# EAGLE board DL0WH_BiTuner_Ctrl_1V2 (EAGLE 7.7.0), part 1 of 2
DL0WH Antenna BiTuner
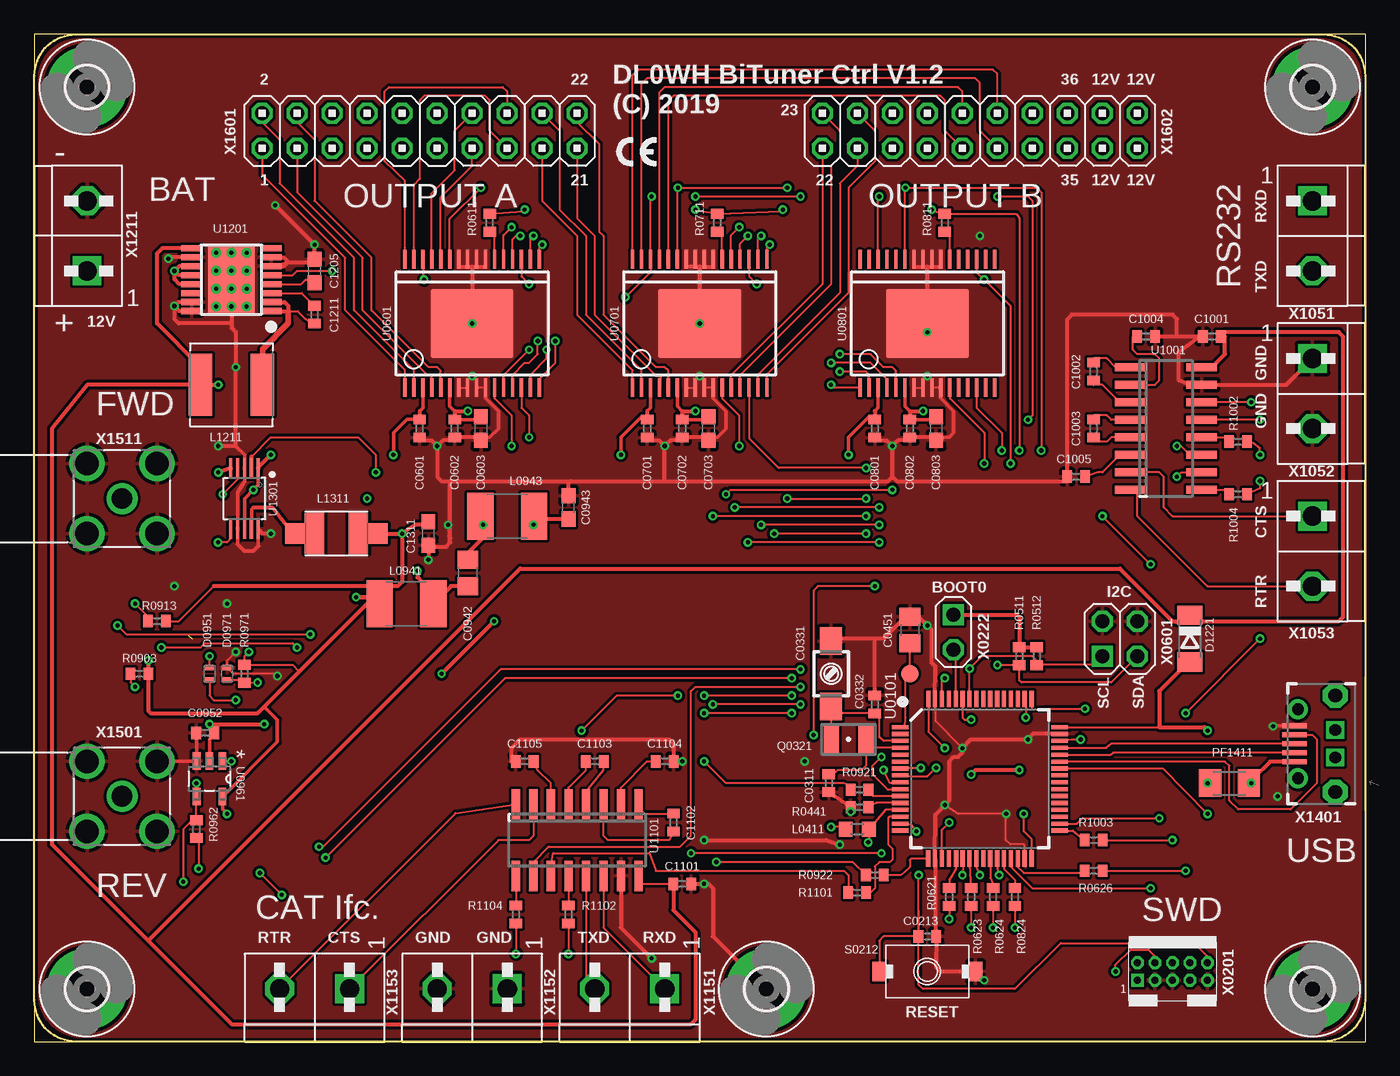
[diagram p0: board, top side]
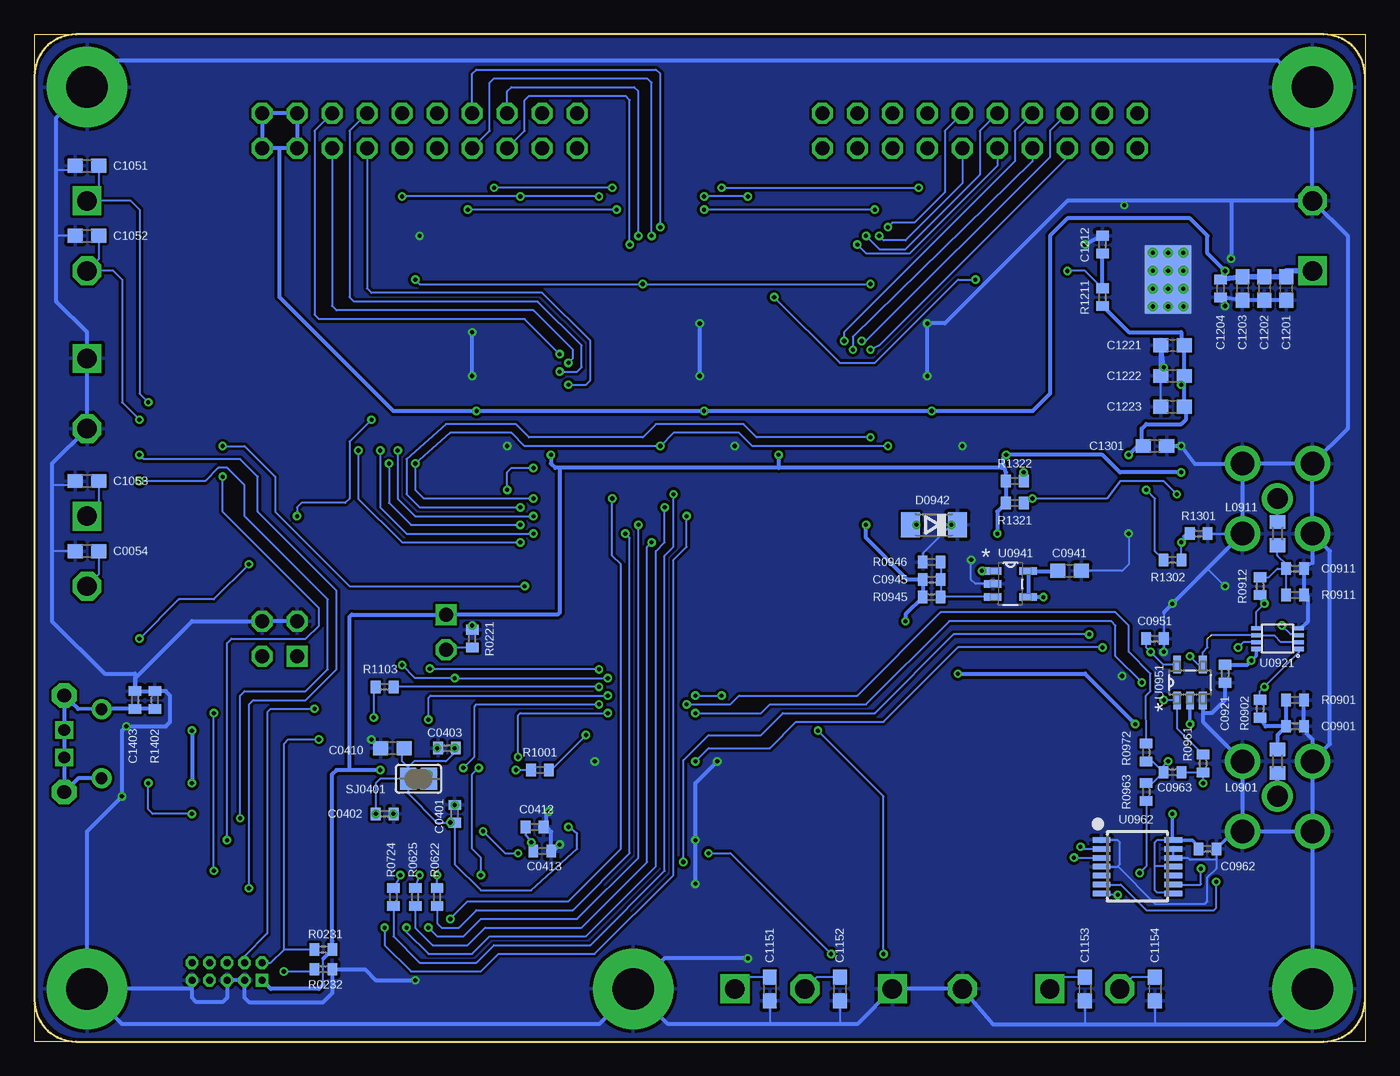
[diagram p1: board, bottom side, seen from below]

Size 96.52 x 73.03 mm. Coordinates in mm from the lower left corner, seen from the top.
Outline: 0,0 96.52,0 96.52,73.03 0,73.03 0,0
Copper layers (1*16): Top 0.035mm / dielectric 1.5mm / Bottom 0.035mm
Design rules "DL0WH_BiTuner_MCU_1V2": minimum track width 6mil, minimum drill 0.3mm, track to track 8mil, track to pad 8mil, pad to pad 6mil, via to via 8mil, smd to smd 0mil, copper to edge 10mil, drill to drill 10mil, minimum pad ring 8mil, minimum via ring 6mil, stop-mask expansion 2mil, vias tented up to drill 25mil, thermal gap 10mil
Net classes: 1 pwr_relay: width 1.5 mm, clearance 0.5 mm; 2 pwr_ttl: width 0.75 mm, clearance 0.5 mm; 3 usb_pair: width 0.254 mm, clearance 0.152 mm; 4 pwrA5: width 0.4 mm; 5 single50R: width 0.838 mm, clearance 0.152 mm; 6 mil6_nofill: width 0.152 mm, clearance 0.254 mm
Milling: 8 lines

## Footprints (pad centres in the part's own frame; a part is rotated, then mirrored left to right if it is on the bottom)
C0603 = smd 1.1 x 1: 1 -0.85,0; 2 0.85,0
C0402 = smd 0.7 x 0.9: 1 -0.65,0; 2 0.65,0
3MM2_X_2MM5 = smd 2 x 1.6: + -2.365,0; - 2.365,0
C0805 = smd 1.3 x 1.5: 1 -0.95,0; 2 0.95,0
SOD80C = smd 1.4 x 1.8: A 1.7,0; C -1.7,0
SOD923 = smd 0.4 x 0.6: A 0.45,0; C -0.45,0
3,0-PAD = drill 3 pad 5.842: B3,0 0,0
L0603 = smd 1 x 1.1: 1 -0.85,0; 2 0.85,0
L1812 = smd 1.9 x 3.4: 1 -1.95,0; 2 1.95,0
L_6.00MM_X_6.00MM = smd 1.7 x 4.5: 1 -2.25,0; 2 2.25,0
L_4.50MM_X_3.20MM = smd 1.5 x 3: 1 -1.6,0; 2 1.6,0 | smd 2 x 1.5: 3 -2.75,0; 4 2.75,0
M1206 = smd 1.6 x 2: 1 -1.4,0; 2 1.4,0
ABS07 = smd 1.1 x 1.9: 1 -1.25,0; 2 1.25,0
R0402 = smd 0.7 x 0.9: 1 -0.65,0; 2 0.65,0
KSR223G_SMD_1POL = smd 1 x 1.4: 1 -3.5,0; 2 3.5,0
SJ = smd 1.168 x 1.6: 1 -0.762,0; 2 0.762,0
B1,27 = smd 1.27 x 1.27: TP 0,0
LQFP64 = smd 1.2 x 0.3: 1 -5.775,3.75; 2 -5.775,3.25; 3 -5.775,2.75; 4 -5.775,2.25; 5 -5.775,1.75; 6 -5.775,1.25; 7 -5.775,0.75; 8 -5.775,0.25; 9 -5.775,-0.25; 10 -5.775,-0.75; 11 -5.775,-1.25; 12 -5.775,-1.75; 13 -5.775,-2.25; 14 -5.775,-2.75; 15 -5.775,-3.25; 16 -5.775,-3.75; 33 5.775,-3.75; 34 5.775,-3.25; 35 5.775,-2.75; 36 5.775,-2.25; 37 5.775,-1.75; 38 5.775,-1.25; 39 5.775,-0.75; 40 5.775,-0.25; 41 5.775,0.25; 42 5.775,0.75; 43 5.775,1.25; 44 5.775,1.75; 45 5.775,2.25; 46 5.775,2.75; 47 5.775,3.25; 48 5.775,3.75 | smd 0.3 x 1.2: 17 -3.75,-5.775; 18 -3.25,-5.775; 19 -2.75,-5.775; 20 -2.25,-5.775; 21 -1.725,-5.775; 22 -1.25,-5.775; 23 -0.75,-5.775; 24 -0.25,-5.775; 25 0.25,-5.775; 26 0.75,-5.775; 27 1.25,-5.775; 28 1.75,-5.775; 29 2.25,-5.775; 30 2.75,-5.775; 31 3.25,-5.775; 32 3.75,-5.775; 49 3.75,5.775; 50 3.25,5.775; 51 2.75,5.775; 52 2.25,5.775; 53 1.75,5.775; 54 1.25,5.775; 55 0.75,5.775; 56 0.25,5.775; 57 -0.25,5.775; 58 -0.75,5.775; 59 -1.25,5.775; 60 -1.75,5.775; 61 -2.25,5.775; 62 -2.75,5.775; 63 -3.25,5.775; 64 -3.725,5.775
SOICW32 = smd 0.25 x 1.3: 1 -4.875,-4.65; 2 -4.225,-4.65; 3 -3.575,-4.65; 4 -2.925,-4.65; 5 -2.275,-4.65; 6 -1.625,-4.65; 7 -0.975,-4.65; 8 -0.325,-4.65; 9 0.325,-4.65; 10 0.975,-4.65; 11 1.625,-4.65; 12 2.275,-4.65; 13 2.925,-4.65; 14 3.575,-4.65; 15 4.225,-4.65; 16 4.875,-4.65; 17 4.875,4.65; 18 4.225,4.65; 19 3.575,4.65; 20 2.925,4.65; 21 2.275,4.65; 22 1.625,4.65; 23 0.975,4.65; 24 0.325,4.65; 25 -0.325,4.65; 26 -0.975,4.65; 27 -1.625,4.65; 28 -2.275,4.65; 29 -2.925,4.65; 30 -3.575,4.65; 31 -4.225,4.65; 32 -4.875,4.65 | smd 6 x 5: 33 0,0
R-PDSO-G8 = smd 0.25 x 0.75: 1 -0.75,-1.55; 2 -0.25,-1.55; 3 0.25,-1.55; 4 0.75,-1.55; 5 0.75,1.55; 6 0.25,1.55; 7 -0.25,1.55; 8 -0.75,1.55
SOT95P280X145-5N = smd 1.27 x 0.559: 1 -1.295,0.94; 2 -1.295,0; 3 -1.295,-0.94; 4 1.295,-0.94; 5 1.295,0.94
SOT-23-5 = smd 1.27 x 0.559: 1 -1.295,0.94; 2 -1.295,0; 3 -1.295,-0.94; 4 1.295,-0.94; 5 1.295,0.94
TSSOP14 = smd 0.4 x 1.3: 1 -1.925,-2.6; 2 -1.275,-2.6; 3 -0.625,-2.6; 4 0.025,-2.6; 5 0.675,-2.6; 6 1.325,-2.6; 7 1.975,-2.6; 8 1.975,2.6; 9 1.325,2.6; 10 0.675,2.6; 11 0.025,2.6; 12 -0.625,2.6; 13 -1.275,2.6; 14 -1.925,2.6
SOIC16N = smd 0.6 x 2.2: 1 -4.445,-2.6; 2 -3.175,-2.6; 3 -1.905,-2.6; 4 -0.635,-2.6; 5 0.635,-2.6; 6 1.905,-2.6; 7 3.175,-2.6; 8 4.445,-2.6; 9 4.445,2.6; 10 3.175,2.6; 11 1.905,2.6; 12 0.635,2.6; 13 -0.635,2.6; 14 -1.905,2.6; 15 -3.175,2.6; 16 -4.445,2.6
HTSSOP16 = smd 0.45 x 1.5: 1 -2.275,-2.9; 2 -1.625,-2.9; 3 -0.975,-2.9; 4 -0.325,-2.9; 5 0.325,-2.9; 6 0.975,-2.9; 7 1.625,-2.9; 8 2.275,-2.9; 9 2.275,2.9; 10 1.625,2.9; 11 0.975,2.9; 12 0.325,2.9; 13 -0.325,2.9; 14 -0.975,2.9; 15 -1.625,2.9; 16 -2.275,2.9 | drill 0.305 pad 0.61: PAD 0.65,0; PAD3 -0.65,0; PAD4 -1.95,0; PAD5 1.95,0; PAD6 1.95,1.1; PAD7 1.95,-1.1; PAD8 0.65,1.1; PAD9 0.65,-1.1; PAD10 -0.65,1.1; PAD11 -0.65,-1.1; PAD12 -1.95,1.1; PAD13 -1.95,-1.1 | smd 5 x 3.4: PAD1 0,0 | smd 5 x 3.4 bottom: PAD2 0,0
S-PDSO-G10 = smd 0.3 x 1.45: 1 -1,-2.2; 2 -0.5,-2.2; 3 0,-2.2; 4 0.5,-2.2; 5 1,-2.2; 6 1,2.2; 7 0.5,2.2; 8 0,2.2; 9 -0.5,2.2; 10 -1,2.2
2X05_1MM27_SHROUDED_CORTEX_JTAG_SWD = drill 0.5 pad 0.914 square: 1 -2.54,-0.635 | drill 0.5 pad 0.914 octagon: 2 -2.54,0.635; 3 -1.27,-0.635; 4 -1.27,0.635; 5 0,-0.635; 6 0,0.635; 7 1.27,-0.635; 8 1.27,0.635; 9 2.54,-0.635; 10 2.54,0.635
1X02 = drill 1.016 square: 1 0,0 | drill 1.016 octagon: 2 0,2.54
2X02 = drill 1.016 square: 1 -1.27,-1.27 | drill 1.016 octagon: 2 -1.27,1.27; 3 1.27,-1.27; 4 1.27,1.27
WIRE-TO-BOARD_5MM08_1X02 = drill 1.4 square: 1 0,2.54 | drill 1.4 octagon: 2 0,-2.54
USB-B-MICRO-SMD_MOLEX-105017-0001 = smd 0.35 x 1.8: D+ 0,4.4; D- -0.65,4.4; GND 1.3,4.4; ID 0.65,4.4; VBUS -1.3,4.4 | drill 0.85 pad 1.45: JSHIELD -2.5,4.15; JSHIELD@2 2.5,4.15 | drill 1 pad 1.8 octagon: JSHIELD@3 -3.5,1.45; JSHIELD@6 3.5,1.45 | drill 0.85 square: JSHIELD@4 -1,1.45; JSHIELD@5 1,1.45
SMA_SMT_AMPHENOL_901-143 = drill 1.499: 1 0,0 | drill 1.702: 2 -2.54,2.54; 3 -2.54,-2.54; 4 2.54,-2.54; 5 2.54,2.54
2X10 = drill 1.016 octagon: 1 -11.43,-1.27; 2 -11.43,1.27; 3 -8.89,-1.27; 4 -8.89,1.27; 5 -6.35,-1.27; 6 -6.35,1.27; 7 -3.81,-1.27; 8 -3.81,1.27; 9 -1.27,-1.27; 10 -1.27,1.27; 11 1.27,-1.27; 12 1.27,1.27; 13 3.81,-1.27; 14 3.81,1.27; 15 6.35,-1.27; 16 6.35,1.27; 17 8.89,-1.27; 18 8.89,1.27; 19 11.43,-1.27; 20 11.43,1.27

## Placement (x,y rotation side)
C0054  10nF  [C0603]  92.71,35.56 180 bottom
C0213  100nF  [C0402]  64.77,7.62 0 top
C0311  22pF  [C0402]  57.63,18.73 270 top
C0331  JR200  [3MM2_X_2MM5]  57.78,26.67 270 top
C0332  18pF  [C0402]  60.96,24.45 90 top
C0401  100nF  [C0402]  66.04,16.51 90 bottom
C0402  100nF  [C0402]  71.12,16.51 0 bottom
C0403  100nF  [C0402]  66.6,21.27 180 bottom
C0410  4.7uF  [C0603]  70.56,21.27 180 bottom
C0412  10nF  [C0402]  60.25,15.56 0 bottom
C0413  1uF  [C0402]  59.69,13.81 0 bottom
C0451  47uF  [C0805]  63.5,29.84 90 top
C0601  100nF  [C0402]  27.94,44.45 90 top
C0602  100nF  [C0402]  30.48,44.45 270 top
C0603  22uF  [C0603]  32.38,44.45 270 top
C0701  100nF  [C0402]  44.45,44.45 90 top
C0702  100nF  [C0402]  46.99,44.45 270 top
C0703  22uF  [C0603]  48.9,44.45 270 top
C0801  100nF  [C0402]  60.96,44.45 90 top
C0802  100nF  [C0402]  63.5,44.45 270 top
C0803  22uF  [C0603]  65.41,44.45 270 top
C0901  1nF  [C0402]  5.08,22.86 0 bottom
C0911  1nF  [C0402]  5.08,34.29 0 bottom
C0921  100nF  [C0402]  10.16,26.67 270 bottom
C0941  22uF  [C0603]  21.43,34.13 0 bottom
C0942  2.2uF  [C0805]  31.43,33.97 90 top
C0943  22uF  [C0603]  38.73,38.73 90 top
C0945  1nF  [C0402]  31.43,33.5 180 bottom
C0951  100nF  [C0402]  15.24,29.21 0 bottom
C0952  100nF  [C0402]  12.38,22.38 180 top
C0962  100nF  [C0402]  11.43,13.97 0 bottom
C0963  100pF  [C0402]  13.97,19.53 180 bottom
C1001  1uF  [C0402]  85.41,51.12 180 top
C1002  1uF  [C0402]  76.83,48.58 270 top
C1003  1uF  [C0402]  76.83,44.45 270 top
C1004  1uF  [C0402]  80.64,51.12 0 top
C1005  1uF  [C0402]  75.56,40.96 180 top
C1051  10nF  [C0603]  92.71,63.5 180 bottom
C1052  10nF  [C0603]  92.71,58.42 180 bottom
C1053  10nF  [C0603]  92.71,40.64 180 bottom
C1101  1uF  [C0402]  46.99,11.43 0 top
C1102  1uF  [C0402]  46.35,15.88 270 top
C1103  1uF  [C0402]  40.64,20.32 180 top
C1104  1uF  [C0402]  45.72,20.32 0 top
C1105  1uF  [C0402]  35.56,20.32 180 top
C1151  10nF  [C0603]  43.18,3.81 270 bottom
C1152  10nF  [C0603]  38.1,3.81 270 bottom
C1153  10nF  [C0603]  20.32,3.81 270 bottom
C1154  10nF  [C0603]  15.24,3.81 270 bottom
C1201  10uF  [C0603]  5.71,54.61 270 bottom
C1202  10uF  [C0603]  7.3,54.61 270 bottom
C1203  10uF  [C0603]  8.89,54.61 270 bottom
C1204  10nF  [C0402]  10.48,54.61 270 bottom
C1205  3.3uF  [C0603]  20.32,55.88 270 top
C1211  0.47uF  [C0402]  20.32,52.7 90 top
C1212  100nF  [C0402]  19.05,57.78 90 bottom
C1221  22uF  [C0603]  13.97,50.48 180 bottom
C1222  22uF  [C0603]  13.97,48.26 180 bottom
C1223  22uF  [C0603]  13.97,46.04 180 bottom
C1301  22uF  [C0603]  15.24,43.18 0 bottom
C1311  22uF  [C0603]  28.57,36.83 270 top
C1403  1nF  [C0402]  89.22,24.77 270 bottom
D0942  CRS08  [SOD80C]  31.27,37.47 180 bottom
D0951  CMAD6001  [SOD923]  12.7,26.67 90 top
D0971  CMAD6001  [SOD923]  13.97,26.67 270 top
D1221  CRS08  [SOD80C]  83.82,29.21 270 top
H1711  MOUNT-PAD-ROUND3.0  [3,0-PAD]  3.81,3.81 0 top
H1721  MOUNT-PAD-ROUND3.0  [3,0-PAD]  53.09,3.81 0 top
H1731  MOUNT-PAD-ROUND3.0  [3,0-PAD]  92.71,3.81 0 top
H1751  MOUNT-PAD-ROUND3.0  [3,0-PAD]  3.81,69.22 0 top
H1761  MOUNT-PAD-ROUND3.0  [3,0-PAD]  92.71,69.22 0 top
L0411  10uH  [L0603]  59.69,15.4 0 top
L0901  10uH  [L0603]  6.35,20.32 270 bottom
L0911  10uH  [L0603]  6.35,36.83 90 bottom
L0941  20uH  [L1812]  26.99,31.75 180 top
L0943  20uH  [L1812]  34.29,38.1 180 top
L1211  2.2uH  [L_6.00MM_X_6.00MM]  14.29,47.62 0 top
L1311  10uH  [L_4.50MM_X_3.20MM]  21.91,36.83 180 top
PF1411  1.1A/2.2A  [M1206]  86.68,18.73 180 top
Q0321  ABS07-32.768KHZ  [ABS07]  59.05,21.91 180 top
R0221  33kR  [R0402]  64.77,29.21 270 bottom
R0231  220kR  [R0402]  75.56,6.67 0 bottom
R0232  220kR  [R0402]  75.56,5.24 180 bottom
R0441  0R  [R0402]  59.85,16.99 0 top
R0511  1kR  [R0402]  71.44,27.94 90 top
R0512  1kR  [R0402]  72.71,27.94 90 top
R0611  47R  [R0402]  33.02,59.37 270 top
R0621  47R  [R0402]  66.36,10.48 270 top
R0622  0R  [R0402]  67.31,10.48 270 bottom
R0623  47R  [R0402]  67.94,10.48 270 top
R0624  47R  [R0402]  69.53,10.48 270 top
R0625  47R  [R0402]  68.9,10.48 270 bottom
R0626  47R  [R0402]  76.83,12.38 0 top
R0711  47R  [R0402]  49.53,59.37 270 top
R0724  47R  [R0402]  70.48,10.48 270 bottom
R0811  47R  [R0402]  66.04,59.37 270 top
R0824  47R  [R0402]  71.12,10.48 270 top
R0901  1kR  [R0402]  5.08,24.77 180 bottom
R0902  15kR  [R0402]  7.62,24.13 90 bottom
R0903  150kR  [R0402]  7.62,26.67 0 top
R0911  1kR  [R0402]  5.08,32.38 180 bottom
R0912  15kR  [R0402]  7.62,33.02 270 bottom
R0913  150kR  [R0402]  8.89,30.48 0 top
R0921  47R  [R0402]  59.85,18.26 180 top
R0922  47R  [R0402]  60.96,12.06 180 top
R0945  8.2kR  [R0402]  31.43,32.23 180 bottom
R0946  33kR  [R0402]  31.43,34.77 0 bottom
R0961  1kR  [R0402]  11.75,20.16 270 bottom
R0962  1.0kR  [R0402]  11.75,15.4 270 top
R0963  10kR  [R0402]  15.88,18.1 90 bottom
R0971  10kR  [R0402]  15.24,26.67 270 top
R0972  47R  [R0402]  15.88,20.95 90 bottom
R1001  47R  [R0402]  59.85,19.68 0 bottom
R1002  47R  [R0402]  87.31,43.5 180 top
R1003  47R  [R0402]  76.83,14.61 0 top
R1004  47R  [R0402]  87.31,39.69 180 top
R1101  47R  [R0402]  59.69,10.79 180 top
R1102  47R  [R0402]  38.73,9.21 90 top
R1103  47R  [R0402]  71.12,25.72 0 bottom
R1104  47R  [R0402]  34.92,9.21 90 top
R1211  3R  [R0402]  19.05,53.98 270 bottom
R1301  100kR  [R0402]  12.06,36.83 180 bottom
R1302  220kR  [R0402]  13.97,34.92 180 bottom
R1321  1MR  [R0402]  25.4,39.05 180 bottom
R1322  1MR  [R0402]  25.4,40.64 180 bottom
R1402  330kR  [R0402]  87.79,24.77 270 bottom
S0212  KSR223GLFG  [KSR223G_SMD_1POL]  64.77,5.08 180 top
SJ0401  [SJ]  68.66,19.05 180 bottom
TP_VBAT  PTR1B1,27  [B1,27]  63.5,26.67 0 top
U0101  STM32L476RXT_64PIN_LDO  [LQFP64]  68.58,19.05 0 top
U0601  MC33996  [SOICW32]  31.75,52.07 0 top
U0701  MC33996  [SOICW32]  48.26,52.07 0 top
U0801  MC33996  [SOICW32]  64.77,52.07 0 top
U0921  TS5A23166  [R-PDSO-G8]  6.35,29.21 90 bottom
U0941  LM2611  [SOT95P280X145-5N]  25.72,33.18 0 bottom
U0951  OPA354  [SOT-23-5]  12.7,26.04 90 bottom
U0961  OPA354  [SOT-23-5]  12.7,19.05 270 top
U0962  MCP4661-103E-MS  [TSSOP14]  16.51,12.7 270 bottom
U1001  MAX232_SOIC16  [SOIC16N]  82.07,44.45 270 top
U1101  MAX232_SOIC16  [SOIC16N]  39.37,14.61 180 top
U1201  LM53603-Q1  [HTSSOP16]  14.29,55.24 90 top
U1301  TPS62056  [S-PDSO-G10]  15.24,39.37 180 top
X0201  FTSH-105-01-F-D-K  [2X05_1MM27_SHROUDED_CORTEX_JTAG_SWD]  82.55,5.08 0 top
X0222  [1X02]  66.67,30.96 180 top
X0601  [2X02]  78.74,29.21 0 top
X1051  WIRE-TO-BOARD_5MM08_1X02  [WIRE-TO-BOARD_5MM08_1X02]  92.71,58.42 0 top
X1052  WIRE-TO-BOARD_5MM08_1X02  [WIRE-TO-BOARD_5MM08_1X02]  92.71,46.99 0 top
X1053  WIRE-TO-BOARD_5MM08_1X02  [WIRE-TO-BOARD_5MM08_1X02]  92.71,35.56 0 top
X1151  WIRE-TO-BOARD_5MM08_1X02  [WIRE-TO-BOARD_5MM08_1X02]  43.18,3.81 270 top
X1152  WIRE-TO-BOARD_5MM08_1X02  [WIRE-TO-BOARD_5MM08_1X02]  31.75,3.81 270 top
X1153  WIRE-TO-BOARD_5MM08_1X02  [WIRE-TO-BOARD_5MM08_1X02]  20.32,3.81 270 top
X1211  WIRE-TO-BOARD_5MM08_1X02  [WIRE-TO-BOARD_5MM08_1X02]  3.81,58.42 180 top
X1401  MOLEX 105017-0001  [USB-B-MICRO-SMD_MOLEX-105017-0001]  95.81,21.59 90 top
X1501  SMA_SMT_AMPHENOL-901-143  [SMA_SMT_AMPHENOL_901-143]  6.35,17.78 90 top
X1511  SAMTEC SMA-J-P-H-RA-TH1  [SMA_SMT_AMPHENOL_901-143]  6.35,39.37 90 top
X1601  [2X10]  27.94,66.04 0 top
X1602  [2X10]  68.58,66.04 0 top

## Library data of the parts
C0054 C0213 C0311 C0332 C0401-C0403 C0410 C0412 C0413 C0451 C0601-C0603 C0701-C0703 C0801-C0803 C0901 C0911 C0921 C0941-C0943 C0945 C0951 C0952 C0962 C0963 C1001-C1005 C1051-C1053 C1101-C1105 C1151-C1154 C1201-C1205 C1211 C1212 C1221-C1223 C1301 C1311 C1403 L0411 L0901 L0911 L0941 L0943 L1211 L1311 R0221 R0231 R0232 R0441 R0511 R0512 R0611 R0621-R0626 R0711 R0724 R0811 R0824 R0901-R0903 R0911-R0913 R0921 R0922 R0945 R0946 R0961-R0963 R0971 R0972 R1001-R1004 R1101-R1104 R1211 R1301 R1302 R1321 R1322 R1402 = df4iah_rcl
C0331 = df4iah_c-trimm
D0942 D0951 D0971 D1221 = df4iah_diode
H1711 H1721 H1731 H1751 H1761 = df4iah_holes
PF1411 = rcl
Q0321 = df4iah_crystal; FARNELL: 2467865; MANUFACTURER: ABS07-32.768KHZ-1-T
S0212 = df4iah_switch
SJ0401 = df4iah_jumper
TP_VBAT = testpad
U0101 = df4iah_stm32l4
U0601 U0701 U0801 = df4iah_dataconvertion
U0921 = df4iah_sc-switches
U0941 U1201 U1301 = df4iah_powersupply
U0951 U0961 = df4iah_opamp; MPN: OPA354AIDBVT; OC_FARNELL: 1207050; OC_NEWARK: -; PACKAGE: SOT-23-5; SUPPLIER: Texas Instruments
U0962 = df4iah_dig-pot
U1001 U1101 = df4iah_dataconvertion; MF: MAXIM; MPN: MAX232ECDR; OC_FARNELL: 2463694; OC_NEWARK: unknown
X0201 X0222 X0601 X1051-X1053 X1151-X1153 X1211 X1401 X1601 X1602 = df4iah_connector
X1501 X1511 = df4iah_connector; MPN: 901-143; OC_FARNELL: 1461631; OC_NEWARK: 51F3841; PACKAGE: RF/COAXIAL, SMA JACK, R/A, 50OHM, THD; SUPPLIER: Amphenol

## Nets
+3V3: C0601.2 C0701.2 C0801.2 C0921.1 C0941.1 C0951.1 C0962.1 C1311.1 L0941.2 L1311.1 L1311.3 R0231.2 R0511.2 R0512.2 R0903.2 R0913.2 R0971.1 R1321.2 R1322.2 SJ0401.1 U0601.3 U0701.3 U0801.3 U0921.8 U0941.4 U0941.5 U0951.5 U0961.5 U0962.8 U0962.11 U0962.14 U1301.5 X0201.1 X0222.1
+5V: C1001.1 C1101.1 C1221.1 C1222.1 C1223.1 C1301.1 D1221.C L1211.1 R1211.2 R1302.2 U1001.16 U1101.16 U1201.9 U1301.1 U1301.8
+12V: C0602.1 C0603.1 C0702.1 C0703.1 C0802.1 C0803.1 C1201.1 C1202.1 C1203.1 C1204.1 U0601.6 U0701.6 U0801.6 U1201.11 U1201.12 U1201.13 X1211.1 X1602.17 X1602.18 X1602.19 X1602.20
-1V5: C0943.1 C0945.2 C0952.1 L0943.1 R0945.2 U0951.2 U0961.2
CAT_DTE_CTS: C1153.1 U1101.7 X1153.1
CAT_DTE_RTR: C1154.1 U1101.8 X1153.2
CAT_DTE_RXD: C1151.1 U1101.14 X1151.1
CAT_DTE_TXD: C1152.1 U1101.13 X1151.2
CAT_MX_C1N: C1102.2 U1101.3
CAT_MX_C1P: C1102.1 U1101.1
CAT_MX_C2M: C1103.2 U1101.5
CAT_MX_C2P: C1103.1 U1101.4
CAT_MX_VM: C1105.1 U1101.6
CAT_MX_VP: C1104.1 U1101.2
DRV_OUT_3_4: U0801.12
DRV_OUT_3_5: U0801.13
DRV_OUT_3_6: U0801.15
DRV_OUT_3_7: U0801.16
DRV_OUT_3_8: U0801.17
DRV_OUT_3_9: U0801.18
DRV_OUT_3_10: U0801.20
DRV_OUT_3_11: U0801.21
DRV_OUT_3_12: U0801.28
DRV_OUT_3_13: U0801.29
DRV_OUT_3_14: U0801.31
DRV_OUT_3_15: U0801.32
GND: C0054.2 C0213.2 C0311.2 C0331.+ C0332.2 C0401.2 C0402.2 C0403.2 C0410.2 C0412.2 C0413.2 C0451.2 C0601.1 C0602.2 C0603.2 C0701.1 C0702.2 C0703.2 C0801.1 C0802.2 C0803.2 C0901.2 C0911.2 C0921.2 C0941.2 C0943.2 C0951.2 C0952.2 C0962.2 C1001.2 C1004.2 C1005.2 C1051.2 C1052.2 C1053.2 C1101.2 C1104.2 C1105.2 C1151.2 C1152.2 C1153.2 C1154.2 C1201.2 C1202.2 C1203.2 C1204.2 C1205.1 C1212.2 C1221.2 C1222.2 C1223.2 C1301.2 C1311.2 C1403.1 D0942.C D0971.C H1711.B3,0 H1721.B3,0 H1731.B3,0 H1751.B3,0 H1761.B3,0 R0221.1 R0232.1 R0441.1 R0901.1 R0911.1 R0946.1 R1301.1 R1402.1 S0212.1 U0101.18 U0101.31 U0101.47 U0101.63 U0601.7 U0601.8 U0601.9 U0601.10 U0601.23 U0601.24 U0601.25 U0601.26 U0601.33 U0701.7 U0701.8 U0701.9 U0701.10 U0701.23 U0701.24 U0701.25 U0701.26 U0701.33 U0801.7 U0801.8 U0801.9 U0801.10 U0801.23 U0801.24 U0801.25 U0801.26 U0801.33 U0921.4 U0941.2 U0951.3 U0961.3 U0962.1 U0962.4 U0962.12 U0962.13 U1001.15 U1101.15 U1201.6 U1201.7 U1201.10 U1201.15 U1201.16 U1201.PAD U1201.PAD1 U1201.PAD2 U1201.PAD3 U1201.PAD4 U1201.PAD5 U1201.PAD6 U1201.PAD7 U1201.PAD8 U1201.PAD9 U1201.PAD10 U1201.PAD11 U1201.PAD12 U1201.PAD13 U1301.3 U1301.7 U1301.10 X0201.3 X0201.5 X0201.9 X0601.2 X0601.4 X1052.1 X1052.2 X1152.1 X1152.2 X1211.2 X1401.GND X1501.2 X1501.3 X1501.4 X1501.5 X1511.2 X1511.3 X1511.4 X1511.5
LM2611_NFB: C0945.1 R0945.1 R0946.2 U0941.3
LM2611_SW: C0942.1 L0941.1 U0941.1
LM53603_!RESET: U1201.8
LM53603_BIAS: C1212.1 R1211.1 U1201.5
LM53603_CBOOT: C1211.2 U1201.3
LM53603_SW: C1211.1 L1211.2 U1201.1 U1201.2
LM53603_VCC: C1205.2 U1201.4
LM_DA: C0942.2 D0942.A L0943.2
MCU_NRST: C0213.1 S0212.2 U0101.7 X0201.10
MCU_VBAT: C0451.1 TP_VBAT.TP U0101.1
MCU_VDD: C0401.1 C0402.1 C0403.1 C0410.1 L0411.1 SJ0401.2 U0101.19 U0101.32 U0101.64
MCU_VDDA: C0412.1 C0413.1 L0411.2 U0101.13
MCU_VREF_M: R0441.2 U0101.12
MP_CAT_CTS_R: R1103.2 U1101.10
MP_CAT_RTR_R: R1104.2 U1101.9
MP_CAT_RXD_R: R1101.2 U1101.11
MP_CAT_TXD_R: R1102.2 U1101.12
MP_RS_CTS_R [mil6_nofill]: R1003.2 U1001.10
MP_RS_RTR_R: R1004.2 U1001.9
MP_RS_RXD_R [mil6_nofill]: R1001.2 U1001.11
MP_RS_TXD_R: R1002.2 U1001.12
N$12: R0611.2 U0601.22
N$13: R0711.2 U0701.22
N$15: R0811.2 U0801.22
OPA_FB: R0963.1 U0962.7
OPA_PULL: R0962.2 U0962.9
PA0: R1101.1 U0101.14
PA1: R1102.1 U0101.15
PA2: U0101.16
PA3: R0922.1 U0101.17
PA4: U0101.20
PA5: R0621.1 U0101.21
PA6: R0622.1 U0101.22
PA7: R0623.1 U0101.23
PA8: U0101.41
PA9: PF1411.1 U0101.42 X1401.VBUS
PA10: U0101.43 X1401.ID
PA11: U0101.44 X1401.D-
PA12: U0101.45 X1401.D+
PA13: R0231.1 U0101.46 X0201.2
PA14: R0232.2 U0101.49 X0201.4
PA15: R1103.1 U0101.50
PB0: R0624.1 U0101.26
PB1: R0724.1 U0101.27
PB2: R0824.1 U0101.28
PB3: U0101.55
PB4: U0101.56
PB5: U0101.57
PB6: R0512.1 U0101.58 U0962.2 X0601.1
PB7: R1104.1 U0101.59
PB8: U0101.61
PB9: R0511.1 U0101.62 U0962.3 X0601.3
PB10 [mil6_nofill]: R1002.1 U0101.29
PB11: R0626.1 U0101.30
PB12: R1003.1 U0101.33
PB13 [mil6_nofill]: R1004.1 U0101.34
PB14: U0101.35
PB15: U0101.36
PC0 [mil6_nofill]: R0972.2 U0101.8
PC1: R1001.1 U0101.9
PC2 [mil6_nofill]: D0971.A R0971.2 U0101.10
PC3: R0921.1 U0101.11
PC4: R0625.1 U0101.24
PC5: U0101.25
PC6: U0101.37
PC7: U0101.38
PC8: U0101.39
PC9: U0101.40
PC10: U0101.51
PC11: U0101.52
PC12: U0101.53
PC13: U0101.2
PC14_OSC32_IN: C0331.- C0332.1 Q0321.2 U0101.3
PC15_OSC32_OUT: C0311.1 Q0321.1 U0101.4
PD2: U0101.54
PH0: U0101.5
PH1: U0101.6
PH3_BOOT0: R0221.2 U0101.60 X0222.2
RELAY1 [mil6_nofill]: U0601.1 X1601.1
RELAY2 [mil6_nofill]: U0601.2 X1601.2
RELAY3 [mil6_nofill]: U0601.4 X1601.3
RELAY4 [mil6_nofill]: U0601.5 X1601.4
RELAY5 [mil6_nofill]: U0601.12 X1601.5
RELAY6 [mil6_nofill]: U0601.13 X1601.6
RELAY7 [mil6_nofill]: U0601.15 X1601.7
RELAY8 [mil6_nofill]: U0601.16 X1601.8
RELAY9: U0601.17 X1601.9
RELAY10 [mil6_nofill]: U0601.18 X1601.10
RELAY11 [mil6_nofill]: U0601.20 X1601.11
RELAY12 [mil6_nofill]: U0601.21 X1601.12
RELAY13: U0601.28 X1601.13
RELAY14: U0601.29 X1601.14
RELAY15: U0601.31 X1601.15
RELAY16 [mil6_nofill]: U0601.32 X1601.16
RELAY17 [mil6_nofill]: U0701.1 X1601.17
RELAY18 [mil6_nofill]: U0701.2 X1601.18
RELAY19 [mil6_nofill]: U0701.4 X1601.19
RELAY20 [mil6_nofill]: U0701.5 X1601.20
RELAY21 [mil6_nofill]: U0701.12 X1602.1
RELAY22 [mil6_nofill]: U0701.13 X1602.2
RELAY23 [mil6_nofill]: U0701.15 X1602.3
RELAY24 [mil6_nofill]: U0701.16 X1602.4
RELAY25 [mil6_nofill]: U0701.17 X1602.5
RELAY26 [mil6_nofill]: U0701.18 X1602.6
RELAY27 [mil6_nofill]: U0701.20 X1602.7
RELAY28 [mil6_nofill]: U0701.21 X1602.8
RELAY29 [mil6_nofill]: U0701.28 X1602.9
RELAY30 [mil6_nofill]: U0701.29 X1602.10
RELAY31 [mil6_nofill]: U0701.31 X1602.11
RELAY32 [mil6_nofill]: U0701.32 X1602.12
RELAY33 [mil6_nofill]: U0801.1 X1602.13
RELAY34 [mil6_nofill]: U0801.2 X1602.14
RELAY35 [mil6_nofill]: U0801.4 X1602.15
RELAY36 [mil6_nofill]: U0801.5 X1602.16
RM_FWD: L0901.2 X1501.1
RM_REV: L0911.2 X1511.1
RS_DTE_CTS: C1053.1 U1001.7 X1053.1
RS_DTE_RTR: C0054.1 U1001.8 X1053.2
RS_DTE_RXD: C1051.1 U1001.14 X1051.1
RS_DTE_TXD: C1052.1 U1001.13 X1051.2
RS_MX_C1N1: C1002.2 U1001.3
RS_MX_C1P: C1002.1 U1001.1
RS_MX_C2M1: C1003.2 U1001.5
RS_MX_C2P: C1003.1 U1001.4
RS_MX_VM: C1005.1 U1001.6
RS_MX_VP: C1004.1 U1001.2
SPI_DRV_!RST [mil6_nofill]: R0625.2 U0601.27 U0701.27 U0801.27
SPI_DRV_C_!CS [mil6_nofill]: R0724.2 U0701.14
SPI_DRV_EXT_!CS [mil6_nofill]: R0824.2 U0801.14
SPI_DRV_L_!CS [mil6_nofill]: R0624.2 U0601.14
SPI_DRV_PWM [mil6_nofill]: R0626.2 U0601.30 U0701.30 U0801.30
SPI_DRV_SCLK [mil6_nofill]: R0621.2 U0601.11 U0701.11 U0801.11
SPI_DRV_SI [mil6_nofill]: R0623.2 U0601.19 U0701.19 U0801.19
SPI_DRV_SO [mil6_nofill]: R0611.1 R0622.2 R0711.1 R0811.1
SWR_IN_FWD: R0902.2 R0903.1 U0921.1
SWR_IN_FWD_HI: C0901.1 L0901.1 R0901.2 R0902.1
SWR_IN_REV: R0912.2 R0913.1 U0921.5
SWR_IN_REV_HI: C0911.1 L0911.1 R0911.2 R0912.1
SWR_OP1_OUT: D0951.C R0961.1 U0951.1
SWR_OP2_IN: C0963.1 R0961.2 R0962.1 U0961.4 U0962.6
SWR_OP2_OUT: C0963.2 R0963.2 R0972.1 U0961.1
SWR_SEL_FWD [mil6_nofill]: R0921.2 U0921.7
SWR_SEL_PWR: D0951.A U0921.2 U0921.6 U0951.4
SWR_SEL_REV [mil6_nofill]: R0922.2 U0921.3
TPS_LBI: R1301.2 R1302.1 U1301.6
TPS_LBO: R1322.1 U1301.2
TPS_PG: R1321.1 U1301.4
TPS_SW: L1311.2 L1311.4 U1301.9
USB_SHIELD: C1403.2 R1402.2 X1401.JSHIELD X1401.JSHIELD@2 X1401.JSHIELD@3 X1401.JSHIELD@4 X1401.JSHIELD@5 X1401.JSHIELD@6
VDDUSB: D1221.A PF1411.2 U0101.48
